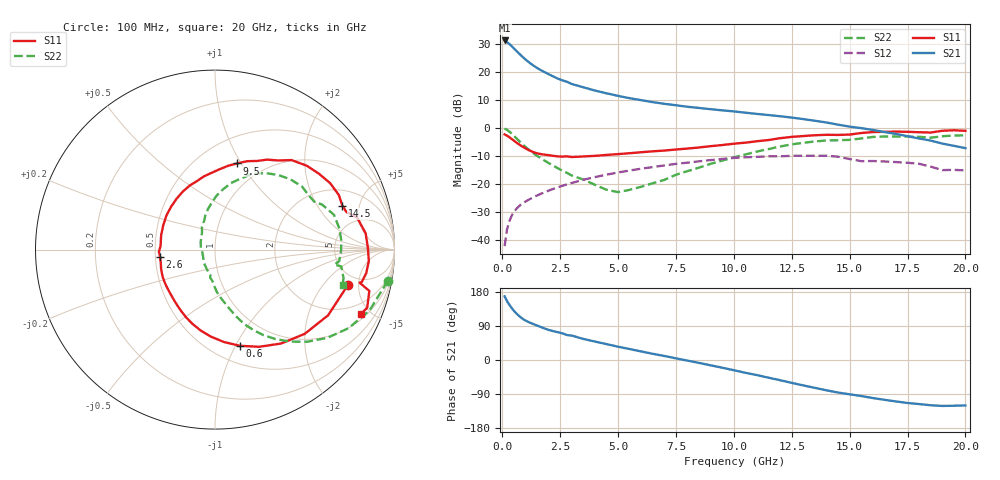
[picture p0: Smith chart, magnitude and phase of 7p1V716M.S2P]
! Infineon Technologies  Discrete & RF Semiconductors
! bfp620
! VCE =  1.7 V,  IC =  16 mA
! Common Emitter S-Parameters:  Sep 2002
# GHz  S  MA  R  50
!  f  S11  S21  S12  S22
! GHz  MAG  ANG  MAG  ANG  MAG  ANG  MAG  ANG
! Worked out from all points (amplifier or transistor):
!   59 points, 100 MHz to 20 GHz, reference 50 ohm
!   highest |S21| = 31.1 dB at 100 MHz (marker M1)
!   |S21| within 3 dB of that: start of sweep to 525.3 MHz
!   unconditionally stable (mu >= 1): 3.652 GHz to 9.999 GHz; 17.14 GHz to end of sweep
!   at 1 GHz: K = 0.62, MSG = 25.3 dB, |S12| = -26.2 dB
!   at 5.5 GHz: K = 1.04, MAG = 11.6 dB, |S12| = -15.1 dB
!   at 20 GHz: K = 1.32, MAG = 0.6 dB, |S12| = -15.1 dB
!   S11 on the Smith chart (normalised r, x): 100 MHz: 3.91, -3.72; 600 MHz: 0.67, -1.04; 2.6 GHz: 0.53, -0.05; 9.5 GHz: 0.76, +0.96; 14.5 GHz: 3.03, +3.39; 20 GHz: 1.29, -4.36
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0.1  0.7666 -14.8  35.87 167.9  0.0079 83.0  0.9781 -10.3
0.2  0.7287 -30.2  33.58 155.9  0.0154 75.3  0.9253 -21.5
0.3  0.6857 -43.2  31.12 146.0  0.0217 70.1  0.8632 -30.5
0.4  0.6397 -54.9  28.54 137.5  0.0272 66.1  0.7954 -38.2
0.5  0.5947 -65.6  26.01 130.0  0.0319 62.9  0.7269 -44.9
0.6  0.5535 -75.5  23.64 123.3  0.0361 60.3  0.6616 -50.8
0.8  0.4854 -92.7  19.6 112.3  0.0431 56.7  0.5485 -60.4
0.9  0.4576 -100.1  17.94 107.9  0.0462 55.4  0.5016 -64.1
1  0.4331 -106.7  16.49 104.2  0.049 54.5  0.4606 -67.3
1.2  0.393 -118.2  14.15 98.3  0.0545 53.1  0.3936 -72.2
1.5  0.3543 -132.8  11.66 91.0  0.0627 51.7  0.32 -77.9
1.9  0.3316 -149.7  9.46 81.5  0.0739 49.9  0.2515 -85.5
2.6  0.3087 -172.4  6.984 70.2  0.0936 46.1  0.1736 -95.2
3.5  0.3106 165.1  5.272 55.6  0.1195 39.7  0.1208 -111.5
5  0.3421 135.5  3.713 35.1  0.1614 27.2  0.0722 -164.7
7  0.3955 104.4  2.681 10.6  0.2153 9.4  0.1193 127.3
9.5  0.496 75.5  2.051 -20.3  0.2805 -16.4  0.2625 93.8
10.5  0.5467 64.6  1.866 -33.8  0.3005 -28.8  0.3375 82.6
13.5  0.7406 30.0  1.34 -73.5  0.3196 -63.9  0.5742 43.1
14.5  0.7505 19.0  1.143 -85.9  0.3076 -78.9  0.6037 30.0
17  0.8594 -4.2  0.781 -109.4  0.2469 -95.3  0.7054 4.1
20  0.8877 -23.9  0.437 -119.9  0.1757 -106.0  0.7372 -15.5
